TYPE "Störungen"
TITLE =Störmeldungen
AUTHOR : dfb
FAMILY : Meld
NAME : 'StörMeld'
VERSION : 0.1


  STRUCT
    Anzahl_Meldeworte : INT  := 37; // AnzahlStörmeldeworte
A : STRUCT //Allgemein Meldung 2001-2016
ST2001_24V_Vers_Zentr : Bool ;  //ST2001: 24V Versorgung Zentrierung gestört
ST2002_24V_Vers : Bool ;  //ST2002: 24V Versorgung gestört
ST2003_230V_Vers : Bool ;  //ST2003: 230V Versorgung gestört
ST2004_Hauptnetz_niO : Bool ;  //ST2004: Hauptstromversorgung ausgefallen
ST2005_Q_Notnetz_niO : Bool ;  //ST2005: Hauptschalter Notstromnetz nicht eingeschaltet
ST2006 : Bool ;  //ST2006:
ST2007_Batt_Fehler_CPU : Bool ;  //ST2007: Batteriefehler Pufferbatterie CPU
ST2008_Profibus : Bool ;  //ST2008: Profibus ist gestört
ST2009_Zentr_Init_niO : Bool ;  //ST2009: Zentrierung ist noch nicht initialisiert! Automatikstart nicht möglich
ST2010_ProdWechsel_n_i_O : Bool ;  //ST2010: Fehler bei Produktwechsel aufgetreten
ST2011 : Bool ;  //ST2011:
ST2012 : Bool ;  //ST2012:
ST2013 : Bool ;  //ST2013:
ST2014 : Bool ;  //ST2014:
ST2015 : Bool ;  //ST2015:
ST2016_KOM_Stoer : Bool ;  //ST2016: Fehler bei Kommunikation (DP/DP-Koppler) aufgetreten
END_STRUCT ;
M : STRUCT //Medien Meldung 2017-2032
ST2017_Gasdr_max : Bool ;  //ST2017: Medien Maximaler Gasdruck ist überschritten
ST2018_Gasdr_min : Bool ;  //ST2018: Medien Minimaler Gasdruck ist unterschritten
ST2019_GDK_niO : Bool ;  //ST2019: Medien Gasdichteprüfung war nicht erfolgreich
ST2020_Pneumatik : Bool ;  //ST2020: Medien Luftdruck Pneumatikversorgung
ST2021 : Bool ;  //ST2021:
ST2022 : Bool ;  //ST2022:
ST2023 : Bool ;  //ST2023:
ST2024 : Bool ;  //ST2024:
ST2025_VBLV_Therm : Bool ;  //ST2025: Verbrennungsluftventilator  Thermistorschutz hat ausgelöst
ST2026_VBLV_MSS : Bool ;  //ST2026: Verbrennungsluftventilator  Motorschutzschalter ist nicht eingeschaltet
ST2027_VBLV_p_Luft : Bool ;  //ST2027: Verbrennungsluftventilator  Fehler bei Druckaufbau Verbrennungsluft
ST2028 : Bool ;  //ST2028:
ST2029_ALV_Therm : Bool ;  //ST2029: Abluftventilator Thermistorschutz hat ausgelöst
ST2030_ALV_MSS : Bool ;  //ST2030: Abluftventilator Motorschutzschalter ist nicht eingeschaltet
ST2031 : Bool ;  //ST2031:
ST2032 : Bool ;  //ST2032:
END_STRUCT ;
Res_03 : STRUCT //Reserve Meldung 2033-2048
ST2033 : Bool ;  //ST2033:
ST2034 : Bool ;  //ST2034:
ST2035 : Bool ;  //ST2035:
ST2036 : Bool ;  //ST2036:
ST2037 : Bool ;  //ST2037:
ST2038 : Bool ;  //ST2038:
ST2039 : Bool ;  //ST2039:
ST2040 : Bool ;  //ST2040:
ST2041 : Bool ;  //ST2041:
ST2042 : Bool ;  //ST2042:
ST2043 : Bool ;  //ST2043:
ST2044 : Bool ;  //ST2044:
ST2045 : Bool ;  //ST2045:
ST2046 : Bool ;  //ST2046:
ST2047 : Bool ;  //ST2047:
ST2048 : Bool ;  //ST2048:
END_STRUCT ;
RG_Allg: STRUCT  //Rollgänge Allgemein Meldung 2049-2064
ST2049_RG02_Stop : Bool ;  //ST2049: RGxy Rollgang 02 steht zu lange
ST2050_RG03_Stop : Bool ;  //ST2050: RGxy Rollgang 03 steht zu lange
ST2051 : Bool ;  //ST2051:
ST2052_PLT_Max_ueberschr : Bool ;  //ST2052: RGxy Zuviele Platinen sind im Ofen! Einfördern wird gesperrt!
ST2053 : Bool ;  //ST2053:
ST2054 : Bool ;  //ST2054:
ST2055 : Bool ;  //ST2055:
ST2056 : Bool ;  //ST2056:
ST2057 : Bool ;  //ST2057:
ST2058 : Bool ;  //ST2058:
ST2059 : Bool ;  //ST2059:
ST2060 : Bool ;  //ST2060:
ST2061 : Bool ;  //ST2061:
ST2062 : Bool ;  //ST2062:
ST2063 : Bool ;  //ST2063:
ST2064 : Bool ;  //ST2064:
END_STRUCT ;
RG01 : STRUCT //Rollgang 01 Meldung 2065-2080
ST2065_RG01_MSS : Bool ;  //ST2065: Rollgang 01 Motorschutzschalter nicht eingeschaltet
ST2066_RG01_SEW_FU : Bool ;  //ST2066: Rollgang 01 Frequenzumrichter gestört
ST2067 : Bool ;  //ST2067:
ST2068_RG01_PB_Stoer : Bool ;  //ST2068: Rollgang 01 FU Profibusstörung
ST2069 : Bool ;  //ST2069:
ST2070 : Bool ;  //ST2070:
ST2071 : Bool ;  //ST2071:
ST2072_RG01_Lfz_Uebers : Bool ;  //ST2072: Rollgang 01 Übersetzen nach Rollgang 02 dauert zu lange
ST2073 : Bool ;  //ST2073:
ST2074 : Bool ;  //ST2074:
ST2075 : Bool ;  //ST2075:
ST2076 : Bool ;  //ST2076:
ST2077 : Bool ;  //ST2077:
ST2078 : Bool ;  //ST2078:
ST2079 : Bool ;  //ST2079:
ST2080 : Bool ;  //ST2080:
END_STRUCT ;
Res_06 : STRUCT //Reserve Meldung 2081-2096
ST2081 : Bool ;  //ST2081:
ST2082 : Bool ;  //ST2082:
ST2083 : Bool ;  //ST2083:
ST2084 : Bool ;  //ST2084:
ST2085 : Bool ;  //ST2085:
ST2086 : Bool ;  //ST2086:
ST2087 : Bool ;  //ST2087:
ST2088 : Bool ;  //ST2088:
ST2089 : Bool ;  //ST2089:
ST2090 : Bool ;  //ST2090:
ST2091 : Bool ;  //ST2091:
ST2092 : Bool ;  //ST2092:
ST2093 : Bool ;  //ST2093:
ST2094 : Bool ;  //ST2094:
ST2095 : Bool ;  //ST2095:
ST2096 : Bool ;  //ST2096:
END_STRUCT ;
RG02 : STRUCT //Rollgang 02 Meldung 2097-2112
ST2097_RG02a_MSS : Bool ;  //ST2097: Rollgang 02a Motorschutzschalter nicht eingeschaltet
ST2098_RG02a_SEW_FU : Bool ;  //ST2098: Rollgang 02a Frequenzumrichter gestört
ST2099 : Bool ;  //ST2099:
ST2100_RG02a_PB_Stoer : Bool ;  //ST2100: Rollgang 02a FU Profibusstörung
ST2101_RG02a_RepSch : Bool ;  //ST2101: Rollgang 02a Reparaturschalter nicht eingeschaltet
ST2102_RG02a_p_Luft : Bool ;  //ST2102: Rollgang 02a Kettenspanner Druckverlust
ST2103_RG02a_Si_Luefter : Bool ;  //ST2103: Rollgang 02a Sicherung Fremdlüfter ausgelöst
ST2104_RG02_Lfz_Schieb_1 : Bool ;  //ST2104: Rollgang 02 Schieber 1 Laufzeitfehler
ST2105_RG02b_MSS : Bool ;  //ST2105: Rollgang 02b Motorschutzschalter nicht eingeschaltet
ST2106_RG02b_SEW_FU : Bool ;  //ST2106: Rollgang 02b Frequenzumrichter gestört
ST2107 : Bool ;  //ST2107:
ST2108_RG02b_PB_Stoer : Bool ;  //ST2108: Rollgang 02b FU Profibusstörung
ST2109_RG02b_RepSch : Bool ;  //ST2109: Rollgang 02b Reparaturschalter nicht eingeschaltet
ST2110_RG02b_p_Luft : Bool ;  //ST2110: Rollgang 02b Kettenspanner Druckverlust
ST2111_RG02b_Si_Luefter : Bool ;  //ST2111: Rollgang 02b Sicherung Fremdlüfter ausgelöst
ST2112_RG02_Lfz_Uebers : Bool ;  //ST2112: Rollgang 02 Übersetzen nach Rollgang 03 dauert zu lange
END_STRUCT ;
Res_08 : STRUCT //Reserve Meldung 2113-2128
ST2113 : Bool ;  //ST2113:
ST2114 : Bool ;  //ST2114:
ST2115 : Bool ;  //ST2115:
ST2116 : Bool ;  //ST2116:
ST2117 : Bool ;  //ST2117:
ST2118 : Bool ;  //ST2118:
ST2119 : Bool ;  //ST2119:
ST2120 : Bool ;  //ST2120:
ST2121 : Bool ;  //ST2121:
ST2122 : Bool ;  //ST2122:
ST2123 : Bool ;  //ST2123:
ST2124 : Bool ;  //ST2124:
ST2125 : Bool ;  //ST2125:
ST2126 : Bool ;  //ST2126:
ST2127 : Bool ;  //ST2127:
ST2128 : Bool ;  //ST2128:
END_STRUCT ;
RG03 : STRUCT //Rollgang 03 Meldung 2129-2144
ST2129_RG03a_MSS : Bool ;  //ST2129: Rollgang 03a Motorschutzschalter nicht eingeschaltet
ST2130_RG03a_SEW_FU : Bool ;  //ST2130: Rollgang 03a Frequenzumrichter gestört
ST2131 : Bool ;  //ST2131:
ST2132_RG03a_PB_Stoer : Bool ;  //ST2132: Rollgang 03a FU Profibusstörung
ST2133_RG03a_RepSch : Bool ;  //ST2133: Rollgang 03a Reparaturschalter nicht eingeschaltet
ST2134 : Bool ;  //ST2134:
ST2135_RG03a_Si_Luefter : Bool ;  //ST2135: Rollgang 03a Sicherung Fremdlüfter ausgelöst
ST2136_RG03_Lfz_Schieb_2 : Bool ;  //ST2136: Rollgang 03 Schieber 2 Laufzeitfehler
ST2137_RG03b_MSS : Bool ;  //ST2137: Rollgang 03b Motorschutzschalter nicht eingeschaltet
ST2138_RG03b_SEW_FU : Bool ;  //ST2138: Rollgang 03b Frequenzumrichter gestört
ST2139 : Bool ;  //ST2139:
ST2140_RG03b_PB_Stoer : Bool ;  //ST2140: Rollgang 03b FU Profibusstörung
ST2141_RG03b_RepSch : Bool ;  //ST2141: Rollgang 03b Reparaturschalter nicht eingeschaltet
ST2142 : Bool ;  //ST2142:
ST2143_RG03b_Si_Luefter : Bool ;  //ST2143: Rollgang 03b Sicherung Fremdlüfter ausgelöst
ST2144_RG03_Lfz_Uebers : Bool ;  //ST2144: Rollgang 03 Uebersetzen nach Rollgang 04 dauert zu lange
END_STRUCT ;
Res_10 : STRUCT //Reserve Meldung 2145-2160
ST2145 : Bool ;  //ST2145:
ST2146 : Bool ;  //ST2146:
ST2147 : Bool ;  //ST2147:
ST2148 : Bool ;  //ST2148:
ST2149 : Bool ;  //ST2149:
ST2150 : Bool ;  //ST2150:
ST2151 : Bool ;  //ST2151:
ST2152 : Bool ;  //ST2152:
ST2153 : Bool ;  //ST2153:
ST2154 : Bool ;  //ST2154:
ST2155 : Bool ;  //ST2155:
ST2156 : Bool ;  //ST2156:
ST2157 : Bool ;  //ST2157:
ST2158 : Bool ;  //ST2158:
ST2159 : Bool ;  //ST2159:
ST2160 : Bool ;  //ST2160:
END_STRUCT ;
RG04 : STRUCT //Rollgang 04 Meldung 2161-2176
ST2161_RG04_MSS : Bool ;  //ST2161: Rollgang 04 Motorschutzschalter nicht eingeschaltet
ST2162_RG04_SEW_FU : Bool ;  //ST2162: Rollgang 04 Frequenzumrichter gestört
ST2163 : Bool ;  //ST2163:
ST2164_RG04_PB_Stoer : Bool ;  //ST2164: Rollgang 04 FU Profibusstörung
ST2165 : Bool ;  //ST2165:
ST2166 : Bool ;  //ST2166:
ST2167_RG04_Sich_Luefter : Bool ;  //ST2167: Rollgang 04 Sicherung Fremdlüfter ausgelöst
ST2168_RG04_BT_niO : Bool ;  //ST2168: Rollgang 04 Platinen n.i.O.
ST2169 : Bool ;  //ST2169:
ST2170 : Bool ;  //ST2170:
ST2171 : Bool ;  //ST2171:
ST2172 : Bool ;  //ST2172:
ST2173 : Bool ;  //ST2173:
ST2174 : Bool ;  //ST2174:
ST2175 : Bool ;  //ST2175:
ST2176 : Bool ;  //ST2176:
END_STRUCT ;
Res_12 : STRUCT //Reserve Meldung 2177-2192
ST2177 : Bool ;  //ST2177:
ST2178 : Bool ;  //ST2178:
ST2179 : Bool ;  //ST2179:
ST2180 : Bool ;  //ST2180:
ST2181 : Bool ;  //ST2181:
ST2182 : Bool ;  //ST2182:
ST2183 : Bool ;  //ST2183:
ST2184 : Bool ;  //ST2184:
ST2185 : Bool ;  //ST2185:
ST2186 : Bool ;  //ST2186:
ST2187 : Bool ;  //ST2187:
ST2188 : Bool ;  //ST2188:
ST2189 : Bool ;  //ST2189:
ST2190 : Bool ;  //ST2190:
ST2191 : Bool ;  //ST2191:
ST2192 : Bool ;  //ST2192:
END_STRUCT ;
Res_13 : STRUCT //Reserve Meldung 2193-2208
ST2193 : Bool ;  //ST2193:
ST2194 : Bool ;  //ST2194:
ST2195 : Bool ;  //ST2195:
ST2196 : Bool ;  //ST2196:
ST2197 : Bool ;  //ST2197:
ST2198 : Bool ;  //ST2198:
ST2199 : Bool ;  //ST2199:
ST2200 : Bool ;  //ST2200:
ST2201 : Bool ;  //ST2201:
ST2202 : Bool ;  //ST2202:
ST2203 : Bool ;  //ST2203:
ST2204 : Bool ;  //ST2204:
ST2205 : Bool ;  //ST2205:
ST2206 : Bool ;  //ST2206:
ST2207 : Bool ;  //ST2207:
ST2208 : Bool ;  //ST2208:
END_STRUCT ;
HZ_Allg : STRUCT //Heizung allgemein Meldung 2209-2224
ST2209_Tempw_Ofen_max : Bool ;  //ST2209: Tempw_Ofen_max  Maximale Ofentemperatur überschritten [Sicherheit
ST2210_BG_TE_ausgef : Bool ;  //ST2210: BG_TE_ausgef  ET200S Temperaturerfassung Heizzonen ist gestört
ST2211 : Bool ;  //ST2211:
ST2212 : Bool ;  //ST2212:
ST2213 : Bool ;  //ST2213:
ST2214 : Bool ;  //ST2214:
ST2215 : Bool ;  //ST2215:
ST2216 : Bool ;  //ST2216:
ST2217 : Bool ;  //ST2217:
ST2218 : Bool ;  //ST2218:
ST2219 : Bool ;  //ST2219:
ST2220 : Bool ;  //ST2220:
ST2221 : Bool ;  //ST2221:
ST2222 : Bool ;  //ST2222:
ST2223 : Bool ;  //ST2223:
ST2224 : Bool ;  //ST2224:
END_STRUCT ;
HZ01 : STRUCT //Heizzone 01 Meldung 2225-2240
ST2225_FB_ReTe_HZ01 : Bool ;  //ST2225: Heizzone 1 Fühlerbruch Regelthermoelement
ST2226_MeUeb_ReTe_HZ01 : Bool ;  //ST2226: Heizzone 1 Messwertüberschreitung Regelthermoelement
ST2227_MeUnt_ReTe_HZ01 : Bool ;  //ST2227: Heizzone 1 Messwertunterschreitung Regelthermoelement
ST2228_MaxTemp_HZ01 : Bool ;  //ST2228: Heizzone 1 Maximaltemperatur überschritten
ST2229_UeberTemp_HZ01 : Bool ;  //ST2229: Heizzone 1 Übertemperatur
ST2230_TempTol_Ueb_HZ01 : Bool ;  //ST2230: Heizzone 1 Temperaturtoleranzüberschreitung
ST2231_TempTol_Unt_HZ01 : Bool ;  //ST2231: Heizzone 1 Temperaturtoleranzunterschreitung
ST2232 : Bool ;  //ST2232:
ST2233 : Bool ;  //ST2233:
ST2234 : Bool ;  //ST2234:
ST2235 : Bool ;  //ST2235:
ST2236 : Bool ;  //ST2236:
ST2237 : Bool ;  //ST2237:
ST2238 : Bool ;  //ST2238:
ST2239 : Bool ;  //ST2239:
ST2240 : Bool ;  //ST2240:
END_STRUCT ;
HZ02 : STRUCT //Heizzone 02 Meldung 2241-2256
ST2241_FB_ReTe_HZ02 : Bool ;  //ST2241: Heizzone 2 Fühlerbruch Regelthermoelement
ST2242_MeUeb_ReTe_HZ02 : Bool ;  //ST2242: Heizzone 2 Messwertüberschreitung Regelthermoelement
ST2243_MeUnt_ReTe_HZ02 : Bool ;  //ST2243: Heizzone 2 Messwertunterschreitung Regelthermoelement
ST2244_MaxTemp_HZ02 : Bool ;  //ST2244: Heizzone 2 Maximaltemperatur überschritten
ST2245_UeberTemp_HZ02 : Bool ;  //ST2245: Heizzone 2 Übertemperatur
ST2246_TempTol_Ueb_HZ02 : Bool ;  //ST2246: Heizzone 2 Temperaturtoleranzüberschreitung
ST2247_TempTol_Unt_HZ02 : Bool ;  //ST2247: Heizzone 2 Temperaturtoleranzunterschreitung
ST2248 : Bool ;  //ST2248:
ST2249 : Bool ;  //ST2249:
ST2250 : Bool ;  //ST2250:
ST2251 : Bool ;  //ST2251:
ST2252 : Bool ;  //ST2252:
ST2253 : Bool ;  //ST2253:
ST2254 : Bool ;  //ST2254:
ST2255 : Bool ;  //ST2255:
ST2256 : Bool ;  //ST2256:
END_STRUCT ;
HZ03 : STRUCT //Heizzone 03 Meldung 2257-2272
ST2257_FB_ReTe_HZ03 : Bool ;  //ST2257: Heizzone 3 Fühlerbruch Regelthermoelement
ST2258_MeUeb_ReTe_HZ03 : Bool ;  //ST2258: Heizzone 3 Messwertüberschreitung Regelthermoelement
ST2259_MeUnt_ReTe_HZ03 : Bool ;  //ST2259: Heizzone 3 Messwertunterschreitung Regelthermoelement
ST2260_MaxTemp_HZ03 : Bool ;  //ST2260: Heizzone 3 Maximaltemperatur überschritten
ST2261_UeberTemp_HZ03 : Bool ;  //ST2261: Heizzone 3 Übertemperatur
ST2262_TempTol_Ueb_HZ03 : Bool ;  //ST2262: Heizzone 3 Temperaturtoleranzüberschreitung
ST2263_TempTol_Unt_HZ03 : Bool ;  //ST2263: Heizzone 3 Temperaturtoleranzunterschreitung
ST2264 : Bool ;  //ST2264:
ST2265 : Bool ;  //ST2265:
ST2266 : Bool ;  //ST2266:
ST2267 : Bool ;  //ST2267:
ST2268 : Bool ;  //ST2268:
ST2269 : Bool ;  //ST2269:
ST2270 : Bool ;  //ST2270:
ST2271 : Bool ;  //ST2271:
ST2272 : Bool ;  //ST2272:
END_STRUCT ;
HZ04 : STRUCT //Heizzone 04 Meldung 2273-2288
ST2273_FB_ReTe_HZ04 : Bool ;  //ST2273: Heizzone 4 Fühlerbruch Regelthermoelement
ST2274_MeUeb_ReTe_HZ04 : Bool ;  //ST2274: Heizzone 4 Messwertüberschreitung Regelthermoelement
ST2275_MeUnt_ReTe_HZ04 : Bool ;  //ST2275: Heizzone 4 Messwertunterschreitung Regelthermoelement
ST2276_MaxTemp_HZ04 : Bool ;  //ST2276: Heizzone 4 Maximaltemperatur überschritten
ST2277_UeberTemp_HZ04 : Bool ;  //ST2277: Heizzone 4 Übertemperatur
ST2278_TempTol_Ueb_HZ04 : Bool ;  //ST2278: Heizzone 4 Temperaturtoleranzüberschreitung
ST2279_TempTol_Unt_HZ04 : Bool ;  //ST2279: Heizzone 4 Temperaturtoleranzunterschreitung
ST2280 : Bool ;  //ST2280:
ST2281 : Bool ;  //ST2281:
ST2282 : Bool ;  //ST2282:
ST2283 : Bool ;  //ST2283:
ST2284 : Bool ;  //ST2284:
ST2285 : Bool ;  //ST2285:
ST2286 : Bool ;  //ST2286:
ST2287 : Bool ;  //ST2287:
ST2288 : Bool ;  //ST2288:
END_STRUCT ;
HZ05 : STRUCT //Heizzone 05 Meldung 2289-2304
ST2289_FB_ReTe_HZ05 : Bool ;  //ST2289: Heizzone 5 Fühlerbruch Regelthermoelement
ST2290_MeUeb_ReTe_HZ05 : Bool ;  //ST2290: Heizzone 5 Messwertüberschreitung Regelthermoelement
ST2291_MeUnt_ReTe_HZ05 : Bool ;  //ST2291: Heizzone 5 Messwertunterschreitung Regelthermoelement
ST2292_MaxTemp_HZ05 : Bool ;  //ST2292: Heizzone 5 Maximaltemperatur überschritten
ST2293_UeberTemp_HZ05 : Bool ;  //ST2293: Heizzone 5 Übertemperatur
ST2294_TempTol_Ueb_HZ05 : Bool ;  //ST2294: Heizzone 5 Temperaturtoleranzüberschreitung
ST2295_TempTol_Unt_HZ05 : Bool ;  //ST2295: Heizzone 5 Temperaturtoleranzunterschreitung
ST2296 : Bool ;  //ST2296:
ST2297 : Bool ;  //ST2297:
ST2298 : Bool ;  //ST2298:
ST2299 : Bool ;  //ST2299:
ST2300 : Bool ;  //ST2300:
ST2301 : Bool ;  //ST2301:
ST2302 : Bool ;  //ST2302:
ST2303 : Bool ;  //ST2303:
ST2304 : Bool ;  //ST2304:
END_STRUCT ;
HZ06 : STRUCT //Heizzone 06 Meldung 2305-2320
ST2305_FB_ReTe_HZ06 : Bool ;  //ST2305: Heizzone 6 Fühlerbruch Regelthermoelement
ST2306_MeUeb_ReTe_HZ06 : Bool ;  //ST2306: Heizzone 6 Messwertüberschreitung Regelthermoelement
ST2307_MeUnt_ReTe_HZ06 : Bool ;  //ST2307: Heizzone 6 Messwertunterschreitung Regelthermoelement
ST2308_MaxTemp_HZ06 : Bool ;  //ST2308: Heizzone 6 Maximaltemperatur überschritten
ST2309_UeberTemp_HZ06 : Bool ;  //ST2309: Heizzone 6 Übertemperatur
ST2310_TempTol_Ueb_HZ06 : Bool ;  //ST2310: Heizzone 6 Temperaturtoleranzüberschreitung
ST2311_TempTol_Unt_HZ06 : Bool ;  //ST2311: Heizzone 6 Temperaturtoleranzunterschreitung
ST2312 : Bool ;  //ST2312:
ST2313 : Bool ;  //ST2313:
ST2314 : Bool ;  //ST2314:
ST2315 : Bool ;  //ST2315:
ST2316 : Bool ;  //ST2316:
ST2317 : Bool ;  //ST2317:
ST2318 : Bool ;  //ST2318:
ST2319 : Bool ;  //ST2319:
ST2320 : Bool ;  //ST2320:
END_STRUCT ;
HZ07 : STRUCT //Heizzone 07 Meldung 2321-2336
ST2321_FB_ReTe_HZ07 : Bool ;  //ST2321: Heizzone 7 Fühlerbruch Regelthermoelement
ST2322_MeUeb_ReTe_HZ07 : Bool ;  //ST2322: Heizzone 7 Messwertüberschreitung Regelthermoelement
ST2323_MeUnt_ReTe_HZ07 : Bool ;  //ST2323: Heizzone 7 Messwertunterschreitung Regelthermoelement
ST2324_MaxTemp_HZ07 : Bool ;  //ST2324: Heizzone 7 Maximaltemperatur überschritten
ST2325_UeberTemp_HZ07 : Bool ;  //ST2325: Heizzone 7 Übertemperatur
ST2326_TempTol_Ueb_HZ07 : Bool ;  //ST2326: Heizzone 7 Temperaturtoleranzüberschreitung
ST2327_TempTol_Unt_HZ07 : Bool ;  //ST2327: Heizzone 7 Temperaturtoleranzunterschreitung
ST2328 : Bool ;  //ST2328:
ST2329 : Bool ;  //ST2329:
ST2330 : Bool ;  //ST2330:
ST2331 : Bool ;  //ST2331:
ST2332 : Bool ;  //ST2332:
ST2333 : Bool ;  //ST2333:
ST2334 : Bool ;  //ST2334:
ST2335 : Bool ;  //ST2335:
ST2336 : Bool ;  //ST2336:
END_STRUCT ;
HZ08 : STRUCT //Heizzone 08 Meldung 2337-2352
ST2337_FB_ReTe_HZ08 : Bool ;  //ST2337: Heizzone 8 Fühlerbruch Regelthermoelement
ST2338_MeUeb_ReTe_HZ08 : Bool ;  //ST2338: Heizzone 8 Messwertüberschreitung Regelthermoelement
ST2339_MeUnt_ReTe_HZ08 : Bool ;  //ST2339: Heizzone 8 Messwertunterschreitung Regelthermoelement
ST2340_MaxTemp_HZ08 : Bool ;  //ST2340: Heizzone 8 Maximaltemperatur überschritten
ST2341_UeberTemp_HZ08 : Bool ;  //ST2341: Heizzone 8 Übertemperatur
ST2342_TempTol_Ueb_HZ08 : Bool ;  //ST2342: Heizzone 8 Temperaturtoleranzüberschreitung
ST2343_TempTol_Unt_HZ08 : Bool ;  //ST2343: Heizzone 8 Temperaturtoleranzunterschreitung
ST2344 : Bool ;  //ST2344:
ST2345 : Bool ;  //ST2345:
ST2346 : Bool ;  //ST2346:
ST2347 : Bool ;  //ST2347:
ST2348 : Bool ;  //ST2348:
ST2349 : Bool ;  //ST2349:
ST2350 : Bool ;  //ST2350:
ST2351 : Bool ;  //ST2351:
ST2352 : Bool ;  //ST2352:
END_STRUCT ;
HZ09 : STRUCT //Heizzone 09 Meldung 2353-2368
ST2353_FB_ReTe_HZ09 : Bool ;  //ST2353: Heizzone 9 Fühlerbruch Regelthermoelement
ST2354_MeUeb_ReTe_HZ09 : Bool ;  //ST2354: Heizzone 9 Messwertüberschreitung Regelthermoelement
ST2355_MeUnt_ReTe_HZ09 : Bool ;  //ST2355: Heizzone 9 Messwertunterschreitung Regelthermoelement
ST2356_MaxTemp_HZ09 : Bool ;  //ST2356: Heizzone 9 Maximaltemperatur überschritten
ST2357_UeberTemp_HZ09 : Bool ;  //ST2357: Heizzone 9 Übertemperatur
ST2358_TempTol_Ueb_HZ09 : Bool ;  //ST2358: Heizzone 9 Temperaturtoleranzüberschreitung
ST2359_TempTol_Unt_HZ09 : Bool ;  //ST2359: Heizzone 9 Temperaturtoleranzunterschreitung
ST2360 : Bool ;  //ST2360:
ST2361 : Bool ;  //ST2361:
ST2362 : Bool ;  //ST2362:
ST2363 : Bool ;  //ST2363:
ST2364 : Bool ;  //ST2364:
ST2365 : Bool ;  //ST2365:
ST2366 : Bool ;  //ST2366:
ST2367 : Bool ;  //ST2367:
ST2368 : Bool ;  //ST2368:
END_STRUCT ;
HZ10 : STRUCT //Heizzone 10 Meldung 2369-2384
ST2369_FB_ReTe_HZ10 : Bool ;  //ST2369: Heizzone 10 Fühlerbruch Regelthermoelement
ST2370_MeUeb_ReTe_HZ10 : Bool ;  //ST2370: Heizzone 10 Messwertüberschreitung Regelthermoelement
ST2371_MeUnt_ReTe_HZ10 : Bool ;  //ST2371: Heizzone 10 Messwertunterschreitung Regelthermoelement
ST2372_MaxTemp_HZ10 : Bool ;  //ST2372: Heizzone 10 Maximaltemperatur überschritten
ST2373_UeberTemp_HZ10 : Bool ;  //ST2373: Heizzone 10 Übertemperatur
ST2374_TempTol_Ueb_HZ10 : Bool ;  //ST2374: Heizzone 10 Temperaturtoleranzüberschreitung
ST2375_TempTol_Unt_HZ10 : Bool ;  //ST2375: Heizzone 10 Temperaturtoleranzunterschreitung
ST2376 : Bool ;  //ST2376:
ST2377 : Bool ;  //ST2377:
ST2378 : Bool ;  //ST2378:
ST2379 : Bool ;  //ST2379:
ST2380 : Bool ;  //ST2380:
ST2381 : Bool ;  //ST2381:
ST2382 : Bool ;  //ST2382:
ST2383 : Bool ;  //ST2383:
ST2384 : Bool ;  //ST2384:
END_STRUCT ;
Res_25 : STRUCT //Reserve Meldung 2385-2400
ST2385 : Bool ;  //ST2385:
ST2386 : Bool ;  //ST2386:
ST2387 : Bool ;  //ST2387:
ST2388 : Bool ;  //ST2388:
ST2389 : Bool ;  //ST2389:
ST2390 : Bool ;  //ST2390:
ST2391 : Bool ;  //ST2391:
ST2392 : Bool ;  //ST2392:
ST2393 : Bool ;  //ST2393:
ST2394 : Bool ;  //ST2394:
ST2395 : Bool ;  //ST2395:
ST2396 : Bool ;  //ST2396:
ST2397 : Bool ;  //ST2397:
ST2398 : Bool ;  //ST2398:
ST2399 : Bool ;  //ST2399:
ST2400 : Bool ;  //ST2400:
END_STRUCT ;
Res_26 : STRUCT //Reserve Meldung 2401-2416
ST2401 : Bool ;  //ST2401:
ST2402 : Bool ;  //ST2402:
ST2403 : Bool ;  //ST2403:
ST2404 : Bool ;  //ST2404:
ST2405 : Bool ;  //ST2405:
ST2406 : Bool ;  //ST2406:
ST2407 : Bool ;  //ST2407:
ST2408 : Bool ;  //ST2408:
ST2409 : Bool ;  //ST2409:
ST2410 : Bool ;  //ST2410:
ST2411 : Bool ;  //ST2411:
ST2412 : Bool ;  //ST2412:
ST2413 : Bool ;  //ST2413:
ST2414 : Bool ;  //ST2414:
ST2415 : Bool ;  //ST2415:
ST2416 : Bool ;  //ST2416:
END_STRUCT ;
Res_27 : STRUCT //Reserve Meldung 2417-2432
ST2417 : Bool ;  //ST2417:
ST2418 : Bool ;  //ST2418:
ST2419 : Bool ;  //ST2419:
ST2420 : Bool ;  //ST2420:
ST2421 : Bool ;  //ST2421:
ST2422 : Bool ;  //ST2422:
ST2423 : Bool ;  //ST2423:
ST2424 : Bool ;  //ST2424:
ST2425 : Bool ;  //ST2425:
ST2426 : Bool ;  //ST2426:
ST2427 : Bool ;  //ST2427:
ST2428 : Bool ;  //ST2428:
ST2429 : Bool ;  //ST2429:
ST2430 : Bool ;  //ST2430:
ST2431 : Bool ;  //ST2431:
ST2432 : Bool ;  //ST2432:
END_STRUCT ;
Res_28: STRUCT //Reserve Meldung 2433-2448
ST2433 : Bool ;  //ST2433:
ST2434 : Bool ;  //ST2434:
ST2435 : Bool ;  //ST2435:
ST2436 : Bool ;  //ST2436:
ST2437 : Bool ;  //ST2437:
ST2438 : Bool ;  //ST2438:
ST2439 : Bool ;  //ST2439:
ST2440 : Bool ;  //ST2440:
ST2441 : Bool ;  //ST2441:
ST2442 : Bool ;  //ST2442:
ST2443 : Bool ;  //ST2443:
ST2444 : Bool ;  //ST2444:
ST2445 : Bool ;  //ST2445:
ST2446 : Bool ;  //ST2446:
ST2447 : Bool ;  //ST2447:
ST2448 : Bool ;  //ST2448:
END_STRUCT ;
Res_29 : STRUCT //Reserve Meldung 2449-2464
ST2449 : Bool ;  //ST2449:
ST2450 : Bool ;  //ST2450:
ST2451 : Bool ;  //ST2451:
ST2452 : Bool ;  //ST2452:
ST2453 : Bool ;  //ST2453:
ST2454 : Bool ;  //ST2454:
ST2455 : Bool ;  //ST2455:
ST2456 : Bool ;  //ST2456:
ST2457 : Bool ;  //ST2457:
ST2458 : Bool ;  //ST2458:
ST2459 : Bool ;  //ST2459:
ST2460 : Bool ;  //ST2460:
ST2461 : Bool ;  //ST2461:
ST2462 : Bool ;  //ST2462:
ST2463 : Bool ;  //ST2463:
ST2464 : Bool ;  //ST2464:
END_STRUCT ;
Res_30 : STRUCT //Reserve Meldung 2465-2480
ST2465 : Bool ;  //ST2465:
ST2466 : Bool ;  //ST2466:
ST2467 : Bool ;  //ST2467:
ST2468 : Bool ;  //ST2468:
ST2469 : Bool ;  //ST2469:
ST2470 : Bool ;  //ST2470:
ST2471 : Bool ;  //ST2471:
ST2472 : Bool ;  //ST2472:
ST2473 : Bool ;  //ST2473:
ST2474 : Bool ;  //ST2474:
ST2475 : Bool ;  //ST2475:
ST2476 : Bool ;  //ST2476:
ST2477 : Bool ;  //ST2477:
ST2478 : Bool ;  //ST2478:
ST2479 : Bool ;  //ST2479:
ST2480 : Bool ;  //ST2480:
END_STRUCT ;
Res_31 : STRUCT //Reserve Meldung 2481-2496
ST2481 : Bool ;  //ST2481:
ST2482 : Bool ;  //ST2482:
ST2483 : Bool ;  //ST2483:
ST2484 : Bool ;  //ST2484:
ST2485 : Bool ;  //ST2485:
ST2486 : Bool ;  //ST2486:
ST2487 : Bool ;  //ST2487:
ST2488 : Bool ;  //ST2488:
ST2489 : Bool ;  //ST2489:
ST2490 : Bool ;  //ST2490:
ST2491 : Bool ;  //ST2491:
ST2492 : Bool ;  //ST2492:
ST2493 : Bool ;  //ST2493:
ST2494 : Bool ;  //ST2494:
ST2495 : Bool ;  //ST2495:
ST2496 : Bool ;  //ST2496:
END_STRUCT ;
Res_32 : STRUCT //Reserve Meldung 2497-2512
ST2497 : Bool ;  //ST2497:
ST2498 : Bool ;  //ST2498:
ST2499 : Bool ;  //ST2499:
ST2500 : Bool ;  //ST2500:
ST2501 : Bool ;  //ST2501:
ST2502 : Bool ;  //ST2502:
ST2503 : Bool ;  //ST2503:
ST2504 : Bool ;  //ST2504:
ST2505 : Bool ;  //ST2505:
ST2506 : Bool ;  //ST2506:
ST2507 : Bool ;  //ST2507:
ST2508 : Bool ;  //ST2508:
ST2509 : Bool ;  //ST2509:
ST2510 : Bool ;  //ST2510:
ST2511 : Bool ;  //ST2511:
ST2512 : Bool ;  //ST2512:
END_STRUCT ;
Res_33 : STRUCT //Reserve Meldung 2513-2528
ST2513 : Bool ;  //ST2513:
ST2514 : Bool ;  //ST2514:
ST2515 : Bool ;  //ST2515:
ST2516 : Bool ;  //ST2516:
ST2517 : Bool ;  //ST2517:
ST2518 : Bool ;  //ST2518:
ST2519 : Bool ;  //ST2519:
ST2520 : Bool ;  //ST2520:
ST2521 : Bool ;  //ST2521:
ST2522 : Bool ;  //ST2522:
ST2523 : Bool ;  //ST2523:
ST2524 : Bool ;  //ST2524:
ST2525 : Bool ;  //ST2525:
ST2526 : Bool ;  //ST2526:
ST2527 : Bool ;  //ST2527:
ST2528 : Bool ;  //ST2528:
END_STRUCT ;
Zentr_1_12_Li_LFZ: STRUCT //Zentrierung 1-12 Links Laufzeit Meldung 2529-2544
ST2529_Finger_1_Li_Lfz : Bool ;  //ST2529: Zentrierung Finger 1 Links Laufzeitfehler
ST2530_Finger_2_Li_Lfz : Bool ;  //ST2530: Zentrierung Finger 2 Links Laufzeitfehler
ST2531_Finger_3_Li_Lfz : Bool ;  //ST2531: Zentrierung Finger 3 Links Laufzeitfehler
ST2532_Finger_4_Li_Lfz : Bool ;  //ST2532: Zentrierung Finger 4 Links Laufzeitfehler
ST2533_Finger_5_Li_Lfz : Bool ;  //ST2533: Zentrierung Finger 5 Links Laufzeitfehler
ST2534_Finger_6_Li_Lfz : Bool ;  //ST2534: Zentrierung Finger 6 Links Laufzeitfehler
ST2535_Finger_7_Li_Lfz : Bool ;  //ST2535: Zentrierung Finger 7 Links Laufzeitfehler
ST2536_Finger_8_Li_Lfz : Bool ;  //ST2536: Zentrierung Finger 8 Links Laufzeitfehler
ST2537_Finger_9_Li_Lfz : Bool ;  //ST2537: Zentrierung Finger 9 Links Laufzeitfehler
ST2538_Finger_10_Li_Lfz : Bool ;  //ST2538: Zentrierung Finger 10 Links Laufzeitfehler
ST2539_Finger_11_Li_Lfz : Bool ;  //ST2539: Zentrierung Finger 11 Links Laufzeitfehler
ST2540_Finger_12_Li_Lfz : Bool ;  //ST2540: Zentrierung Finger 12 Links Laufzeitfehler
ST2541 : Bool ;  //ST2541:
ST2542 : Bool ;  //ST2542:
ST2543 : Bool ;  //ST2543:
ST2544 : Bool ;  //ST2544:
END_STRUCT ;
Zentr_1_12_Re_LFZ: STRUCT //Zentrierung 1-12 Rechts Laufzeit Meldung 2545-2560
ST2545_Finger_1_Re_Lfz : Bool ;  //ST2545: Zentrierung Finger 1 Rechts Laufzeitfehler
ST2546_Finger_2_Re_Lfz : Bool ;  //ST2546: Zentrierung Finger 2 Rechts Laufzeitfehler
ST2547_Finger_3_Re_Lfz : Bool ;  //ST2547: Zentrierung Finger 3 Rechts Laufzeitfehler
ST2548_Finger_4_Re_Lfz : Bool ;  //ST2548: Zentrierung Finger 4 Rechts Laufzeitfehler
ST2549_Finger_5_Re_Lfz : Bool ;  //ST2549: Zentrierung Finger 5 Rechts Laufzeitfehler
ST2550_Finger_6_Re_Lfz : Bool ;  //ST2550: Zentrierung Finger 6 Rechts Laufzeitfehler
ST2551_Finger_7_Re_Lfz : Bool ;  //ST2551: Zentrierung Finger 7 Rechts Laufzeitfehler
ST2552_Finger_8_Re_Lfz : Bool ;  //ST2552: Zentrierung Finger 8 Rechts Laufzeitfehler
ST2553_Finger_9_Re_Lfz : Bool ;  //ST2553: Zentrierung Finger 9 Rechts Laufzeitfehler
ST2554_Finger_10_Re_Lfz : Bool ;  //ST2554: Zentrierung Finger 10 Rechts Laufzeitfehler
ST2555_Finger_11_Re_Lfz : Bool ;  //ST2555: Zentrierung Finger 11 Rechts Laufzeitfehler
ST2556_Finger_12_Re_Lfz : Bool ;  //ST2556: Zentrierung Finger 12 Rechts Laufzeitfehler
ST2557 : Bool ;  //ST2557:
ST2558 : Bool ;  //ST2558:
ST2559 : Bool ;  //ST2559:
ST2560 : Bool ;  //ST2560:
END_STRUCT ;
Zentr_Module: STRUCT //Zentrierung Festo Module Meldung 2561-2576
ST2561_Zentr_PB_1_4_Li : Bool ;  //ST2561: Zentrierung Busstörung Festomodul 1-4 Links
ST2562_Zentr_PB_5_8_Li : Bool ;  //ST2562: Zentrierung Busstörung Festomodul 5-8 Links
ST2563_Zentr_PB_9_12_Li : Bool ;  //ST2563: Zentrierung Busstörung Festomodul 9-12 Links
ST2564_Zentr_PB_1_4_Re : Bool ;  //ST2564: Zentrierung Busstörung Festomodul 1-4 Rechts
ST2565_Zentr_PB_5_8_Re : Bool ;  //ST2565: Zentrierung Busstörung Festomodul 5-8 Rechts
ST2566_Zentr_PB_9_12_Re : Bool ;  //ST2566: Zentrierung Busstörung Festomodul 9-12 Rechts
ST2567_Mod_Li_1_4_Err : Bool ;  //ST2567: Zentrierung Modul 1-4 Links gestört
ST2568_Mod_Li_5_8_Err : Bool ;  //ST2568: Zentrierung Modul 5-8 Links gestört
ST2569_Mod_Li_9_12_Err : Bool ;  //ST2569: Zentrierung Modul 9-12 Links gestört
ST2570_Mod_Re_1_4_Err : Bool ;  //ST2570: Zentrierung Modul 1-4 Rechts gestört
ST2571_Mod_Re_5_8_Err : Bool ;  //ST2571: Zentrierung Modul 5-8 Rechts gestört
ST2572_Mod_Re_9_12_Err : Bool ;  //ST2572: Zentrierung Modul 9-12 Rechts gestört
ST2573 : Bool ;  //ST2573:
ST2574 : Bool ;  //ST2574:
ST2575 : Bool ;  //ST2575:
ST2576 : Bool ;  //ST2576:
END_STRUCT ;
Res_37: STRUCT //Reserve Meldung 2577-2592
ST2577 : Bool ;  //ST2577:
ST2578 : Bool ;  //ST2578:
ST2579 : Bool ;  //ST2579:
ST2580 : Bool ;  //ST2580:
ST2581 : Bool ;  //ST2581:
ST2582 : Bool ;  //ST2582:
ST2583 : Bool ;  //ST2583:
ST2584 : Bool ;  //ST2584:
ST2585 : Bool ;  //ST2585:
ST2586 : Bool ;  //ST2586:
ST2587 : Bool ;  //ST2587:
ST2588 : Bool ;  //ST2588:
ST2589 : Bool ;  //ST2589:
ST2590 : Bool ;  //ST2590:
ST2591 : Bool ;  //ST2591:
ST2592 : Bool ;  //ST2592:
END_STRUCT ;
END_STRUCT ;
END_TYPE
